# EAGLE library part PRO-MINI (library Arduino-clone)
Arduion Pro Mini Clone V1.0 www.betemcu.cu
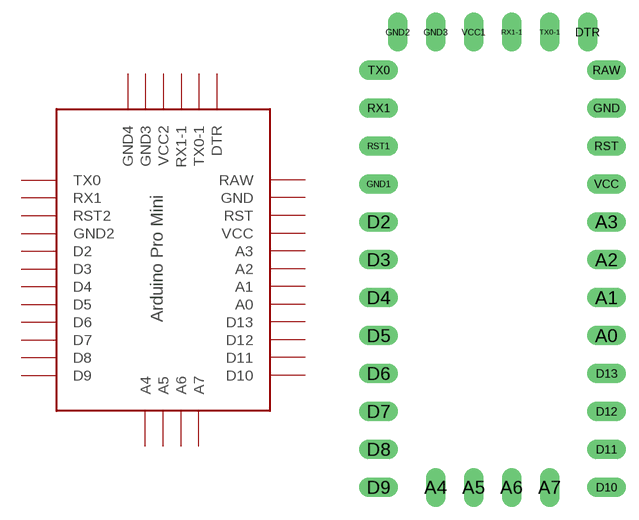
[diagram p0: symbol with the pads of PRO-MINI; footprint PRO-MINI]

Designator prefix -

## PRO-MINI  [PRO-MINI]
A0  A0
A1  A1
A2  A2
A3  A3
A4  A4
A5  A5
A6  A6
A7  A7
D2  D2
D3  D3
D4  D4
D5  D5
D6  D6
D7  D7
D8  D8
D9  D9
D10  D10
D11  D11
D12  D12
D13  D13
DTR  DTR
GND  GND  in
GND1  GND2
GND2  GND4
GND3  GND3
RAW  RAW  pwr
RST  RST
RST1  RST2
RX1  RX1
RX1-1  RX1-1
TX0  TX0
TX0-1  TX0-1
VCC  VCC
VCC1  VCC2

## Footprint PRO-MINI (pad centres in mm)
Arduino Pro Mini Clone
drill 0.8 long: A0 8.89,8.89; A1 8.89,11.43; A2 8.89,13.97; A3 8.89,16.51; A4 -2.54,-1.27; A5 0,-1.27; A6 2.54,-1.27; A7 5.08,-1.27; D2 -6.35,16.51; D3 -6.35,13.97; D4 -6.35,11.43; D5 -6.35,8.89; D6 -6.35,6.35; D7 -6.35,3.81; D8 -6.35,1.27; D9 -6.35,-1.27; D10 8.89,-1.27; D11 8.89,1.27; D12 8.89,3.81; D13 8.89,6.35; DTR 7.62,29.21; GND 8.89,24.13; GND1 -6.35,19.05; GND2 -5.08,29.21; GND3 -2.54,29.21; RAW 8.89,26.67; RST 8.89,21.59; RST1 -6.35,21.59; RX1 -6.35,24.13; RX1-1 2.54,29.21; TX0 -6.35,26.67; TX0-1 5.08,29.21; VCC 8.89,19.05; VCC1 0,29.21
